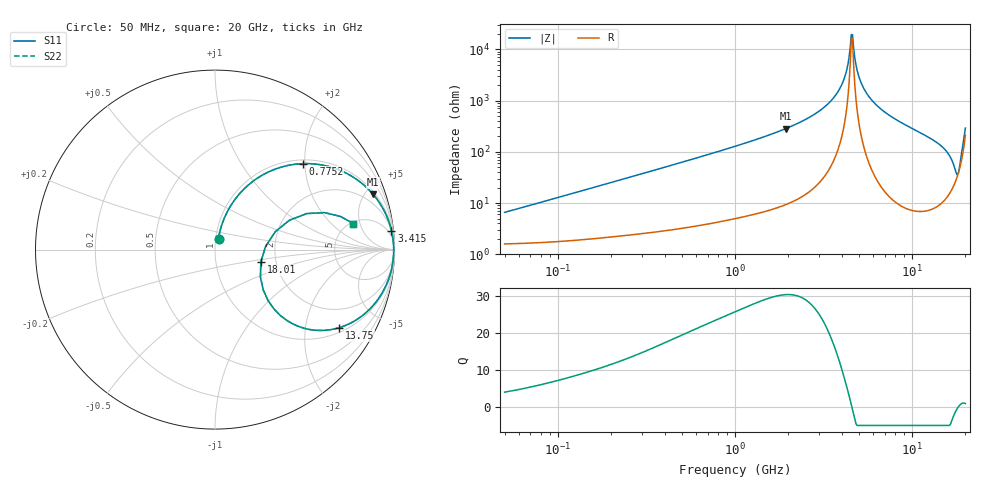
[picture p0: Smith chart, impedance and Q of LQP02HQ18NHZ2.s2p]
!Murata Part Number: LQP02HQ18NHZ2
!These Parameters are Measured in Series Mode Connection
!  o--[Z]--o
!Port1  Port2
!  o-------o
!Freq. Start=50[MHz] Stop=20[GHz], 401[Steps]
# Hz S RI R 50
!Freq.(Hz) S11(Real) S11(Imag) S21(Real) S21(Imag) S12(Real) S12(Imag) S22(Real) S22(Imag)
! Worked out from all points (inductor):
!   401 points, 50 MHz to 20 GHz, reference 50 ohm
!   read as one part in series: L = 20.3 nH near 51.52 MHz
!   highest Q = 30.4 at 1.933 GHz (marker M1), where L = 23.3 nH
!   self-resonance near 4.54 GHz
!   S11 on the Smith chart (normalised r, x): 50 MHz: 1.03, +0.13; 775.2 MHz: 1.08, +1.95; 3.415 GHz: 2, +18; 13.75 GHz: 1.17, -3.05; 18.01 GHz: 1.66, -0.25; 20 GHz: 5.24, +3.96
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5e7  0.0196 0.0618  0.9804 -0.0618  0.9804 -0.0618  0.0196 0.0618
1.364002e8  0.0463 0.1616  0.9537 -0.1616  0.9537 -0.1616  0.0463 0.1616
3.721004e8  0.1918 0.3649  0.8082 -0.3649  0.8082 -0.3649  0.1918 0.3649
7.751977e8  0.4886 0.479  0.5114 -0.479  0.5114 -0.479  0.4886 0.479
1e9  0.6161 0.4673  0.3839 -0.4673  0.3839 -0.4673  0.6161 0.4673
1.932977e9  0.8812 0.3075  0.1188 -0.3075  0.1188 -0.3075  0.8812 0.3075
2.728004e9  0.9561 0.1874  0.0439 -0.1874  0.0439 -0.1874  0.9561 0.1874
3.415248e9  0.983 0.1063  0.017 -0.1063  0.017 -0.1063  0.983 0.1063
4.087748e9  0.9936 0.041  0.00637 -0.041  0.00637 -0.041  0.9936 0.041
4.275624e9  0.9949 0.0246  0.00514 -0.0246  0.00514 -0.0246  0.9949 0.0246
4.472136e9  0.9955 0.00814  0.00449 -0.00814  0.00449 -0.00814  0.9955 0.00814
4.608136e9  0.9956 -0.00286  0.00436 0.00286  0.00436 0.00286  0.9956 -0.00286
4.966507e9  0.9948 -0.0305  0.00517 0.0305  0.00517 0.0305  0.9948 -0.0305
5.352748e9  0.9924 -0.0584  0.00762 0.0584  0.00762 0.0584  0.9924 -0.0584
6.125241e9  0.9836 -0.1094  0.0164 0.1094  0.0164 0.1094  0.9836 -0.1094
7.442007e9  0.9592 -0.1854  0.0408 0.1854  0.0408 0.1854  0.9592 -0.1854
1.375312e10  0.6909 -0.4354  0.3091 0.4354  0.3091 0.4354  0.6909 -0.4354
1.621653e10  0.4351 -0.4148  0.5649 0.4148  0.5649 0.4148  0.4351 -0.4148
1.721783e10  0.2962 -0.2849  0.7038 0.2849  0.7038 0.2849  0.2962 -0.2849
1.800918e10  0.2553 -0.07  0.7447 0.07  0.7447 0.07  0.2553 -0.07
1.912117e10  0.5111 0.2007  0.4889 -0.2007  0.4889 -0.2007  0.5111 0.2007
2e10  0.7715 0.145  0.2285 -0.145  0.2285 -0.145  0.7715 0.145
